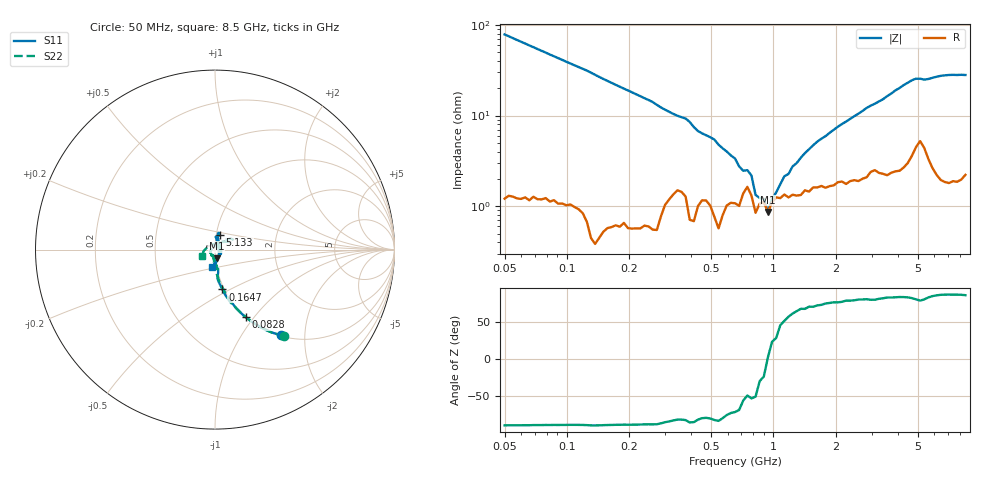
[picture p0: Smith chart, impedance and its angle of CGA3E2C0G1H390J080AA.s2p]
! S-parameter Generated by TDK Corporation
! Copyright(C) 2015 TDK Corporation.
! All Rights Reserved.
! TDK P/N: CGA3E2C0G1H390J080AA (Multilayer Ceramic Chip Capacitors)
! Property: C=39pF
! Size(LxWxT): 1.6x0.8x0.8mm, 0.063x0.031x0.031inches
! Model Type: s2p (Touchstone File Format Version 1.0)
! Frequency: DC=Yes Start=50MHz Stop=8500MHz 114points Log-sweep
! Note:
! Model Generated on Jun. 23, 2015
! Hash(MD5):
! Port Assignments:
!  1 ---| |--- 2
! Applicable Conditions:
!  Temperature = 25 degC
!  DC Bias Voltage = 0 V
!  Small Signal Operation
! Terms and conditions regarding TDK Simulation Models
! (1)This simulation model is being provided solely for informational purposes. Please refer to the specifications of the products in terms of detailed characteristics of such products.
! (2)In no event shall TDK Corporation of any of its subsidiaries be liable for any loss or damage arising, directly or indirectly,
!  From any information contained in this simulation model, including, but not limited to loss or damages arising from any inaccuracies, omissions or errors in connection with such information.
! (3)Any and all copyrights on this simulation model are owned by TDK Corporation.
!  Duplication or redistribution of this simulation model without prior written permission from TDK Corporation is prohibited.
! (4)This simulation model is subject to any modification or change without any prior notice.
! (5)Neither TDK Corporation nor any of its subsidiaries shall make any warranty, express or implied,
!  Including but not limited to the correctness, implied warranties of merchantability and fitness for a particular purpose with respect to this simulation models.
! (6)The use of this simulation model shall be deemed to have consented to the terms and conditions hereof.
# MHz S MA R 50
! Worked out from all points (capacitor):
!   113 points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, 50 MHz to 8.5 GHz, reference 50 ohm
!   read as one part in series: C = 40.6 pF near 50 MHz
!   lowest |Z| = 866 mohm at 940.8 MHz (marker M1)
!   series resonance near 938.2 MHz, so ESL is about 710 pH
!   S11 on the Smith chart (normalised r, x): 50 MHz: 1.01, -1.52; 82.8 MHz: 1.00, -0.91; 164.7 MHz: 0.98, -0.46; 5.133 GHz: 1.04, +0.17; 8.5 GHz: 0.95, -0.18
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50  0.6035 -52.4  0.7772 37.4  0.7776 37.4  0.6189 -51.4
82.80031  0.4134 -65.7  0.8879 24.6  0.8864 24.6  0.4345 -64.1
119.495  0.3045 -72.8  0.9322 17.5  0.9322 17.6  0.3219 -72.2
164.7224  0.2258 -79.5  0.9579 12.3  0.9576 12.3  0.2349 -77.5
285.5811  0.1423 -83.8  0.974 6.0  0.974 6.1  0.1277 -85.5
472.9241  0.07569 -88.4  0.9762 1.9  0.976 2.0  0.0896 -84.7
651.9202  0.06798 -86.5  0.976 -0.1  0.9748 -0.1  0.05932 -96.4
940.8324  0.0502 -79.8  0.9816 -2.6  0.9791 -2.6  0.04109 -112.4
1357.782  0.04433 -63.9  0.9762 -5.4  0.9758 -5.5  0.02988 -130.5
1558.024  0.04081 -54.2  0.9711 -6.8  0.9713 -6.7  0.03288 -133.8
2354.001  0.03674 -19.8  0.9673 -10.9  0.9678 -11.0  0.02801 -162.7
3099.524  0.03675 25.0  0.9606 -14.4  0.9596 -14.4  0.01083 118.3
3244.963  0.03224 39.1  0.961 -15.1  0.9601 -15.1  0.0157 87.6
3397.226  0.03662 45.1  0.9637 -15.9  0.9623 -15.8  0.01834 71.4
3723.522  0.04846 66.4  0.9612 -17.5  0.9605 -17.5  0.04 53.4
4272.658  0.08099 79.3  0.9527 -20.4  0.9538 -20.4  0.07942 43.4
5132.831  0.08594 71.7  0.9256 -23.7  0.9266 -23.6  0.1135 23.9
6455.51  0.05224 78.1  0.9549 -29.3  0.9537 -29.2  0.06012 44.9
7075.547  0.02042 11.1  0.9544 -32.5  0.9563 -32.2  0.03309 88.2
7407.553  0.03213 -45.8  0.955 -34.0  0.9548 -34.0  0.03224 132.7
7755.137  0.05448 -74.1  0.9531 -35.8  0.9529 -35.6  0.04651 167.3
8500  0.09576 -98.7  0.9484 -39.6  0.9484 -39.5  0.08139 -154.7
